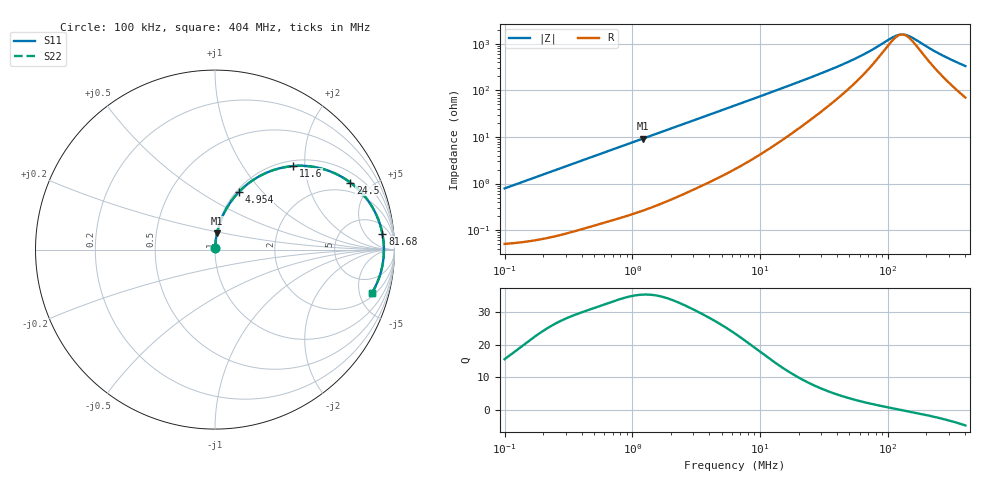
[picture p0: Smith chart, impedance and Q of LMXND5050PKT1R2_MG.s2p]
! LMXND5050PKT1R2_MG  S-PARAMETER MODEL  ( General Type )
! Model Generated by TAIYO YUDEN Corporation (http://www.ty-top.com)
! Version 1.0
! TAIYO YUDEN Control No. 191023NI43SB-FBB
! Copyright(c) 2019 TAIYO YUDEN CO.,LTD. All Rights Reserved.
! Product Description (link to TY-COMPAS)
! https://ds.yuden.co.jp/TYCOMPAS/or/detail?pn=LMXND5050PKT1R2NMG&u=M
! Products Name : Inductors
! Characteristics :
!  Inductance : 1.2 uH , SRF(min) : 86 MHz , DC Resistance(max) : 0.054 Ohm
!  Rated Current : Saturation :3800 mA , Temp Rise : 2400 mA
!  Case Size : 4.9 x 4.9 / 0.193 x 0.193 [mm/inch] , Thickness : 1.4 / 0.055 [mm/inch]
!  (Conditions: Temperature = 25 degC , DC Bias Current/Voltage = 0A / 0V)
! External Node Assignments :
!  1  o---GGG---o  2
! GND o---------o GND
! Frequency Range : 0.1MHz  -  403.964729MHz  [ 402 STEP ]
# MHz S RI R 50
! Freq[MHz].  S11 Real  S11 Imag  S21 Real  S21 Imag  S12 Real  S12 Imag  S22 Real  S22 Imag
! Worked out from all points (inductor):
!   401 points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, 100 kHz to 404 MHz, reference 50 ohm
!   read as one part in series: L = 1.25 uH near 104.2 kHz
!   highest Q = 35.3 at 1.208 MHz (marker M1), where L = 1.22 uH
!   self-resonance near 129.2 MHz
!   S11 on the Smith chart (normalised r, x): 100 kHz: 1.00, +0.02; 4.954 MHz: 1.03, +0.74; 11.6 MHz: 1.11, +1.74; 24.5 MHz: 1.46, +3.73; 81.68 MHz: 10, +14; 404 MHz: 2.41, -6.56
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0.1  0.000565 0.00784  0.9994 -0.00784  0.9994 -0.00784  0.000565 0.00784
0.401849  0.00201 0.0311  0.998 -0.0311  0.998 -0.0311  0.00201 0.0311
1.207544  0.011 0.091  0.989 -0.091  0.989 -0.091  0.011 0.091
1.614823  0.0182 0.1202  0.9818 -0.1202  0.9818 -0.1202  0.0182 0.1202
3.073383  0.0575 0.217  0.9425 -0.217  0.9425 -0.217  0.0575 0.217
4.95429  0.131 0.3188  0.869 -0.3188  0.869 -0.3188  0.131 0.3188
6.355822  0.1954 0.3757  0.8046 -0.3757  0.8046 -0.3757  0.1954 0.3757
8.859831  0.3151 0.4394  0.6849 -0.4394  0.6849 -0.4394  0.3151 0.4394
11.60464  0.4357 0.4655  0.5643 -0.4655  0.5643 -0.4655  0.4357 0.4655
16.51586  0.6007 0.4495  0.3993 -0.4495  0.3993 -0.4495  0.6007 0.4495
24.50206  0.754 0.3738  0.246 -0.3738  0.246 -0.3738  0.754 0.3738
25.54079  0.767 0.3637  0.233 -0.3637  0.233 -0.3637  0.767 0.3637
34.87162  0.8451 0.2835  0.1549 -0.2835  0.1549 -0.2835  0.8451 0.2835
48.61003  0.8962 0.1998  0.1038 -0.1998  0.1038 -0.1998  0.8962 0.1998
63.66959  0.9202 0.1382  0.0798 -0.1382  0.0798 -0.1382  0.9202 0.1382
81.68124  0.933 0.0866  0.067 -0.0866  0.067 -0.0866  0.933 0.0866
102.6353  0.9391 0.0426  0.0609 -0.0426  0.0609 -0.0426  0.9391 0.0426
113.8613  0.9405 0.0233  0.0595 -0.0233  0.0595 -0.0233  0.9405 0.0233
123.7199  0.941 0.00795  0.059 -0.00795  0.059 -0.00795  0.941 0.00795
143.0706  0.9407 -0.0188  0.0593 0.0188  0.0593 0.0188  0.9407 -0.0188
255.8554  0.922 -0.133  0.078 0.133  0.078 0.133  0.922 -0.133
403.9647  0.8752 -0.2402  0.1248 0.2402  0.1248 0.2402  0.8752 -0.2402
